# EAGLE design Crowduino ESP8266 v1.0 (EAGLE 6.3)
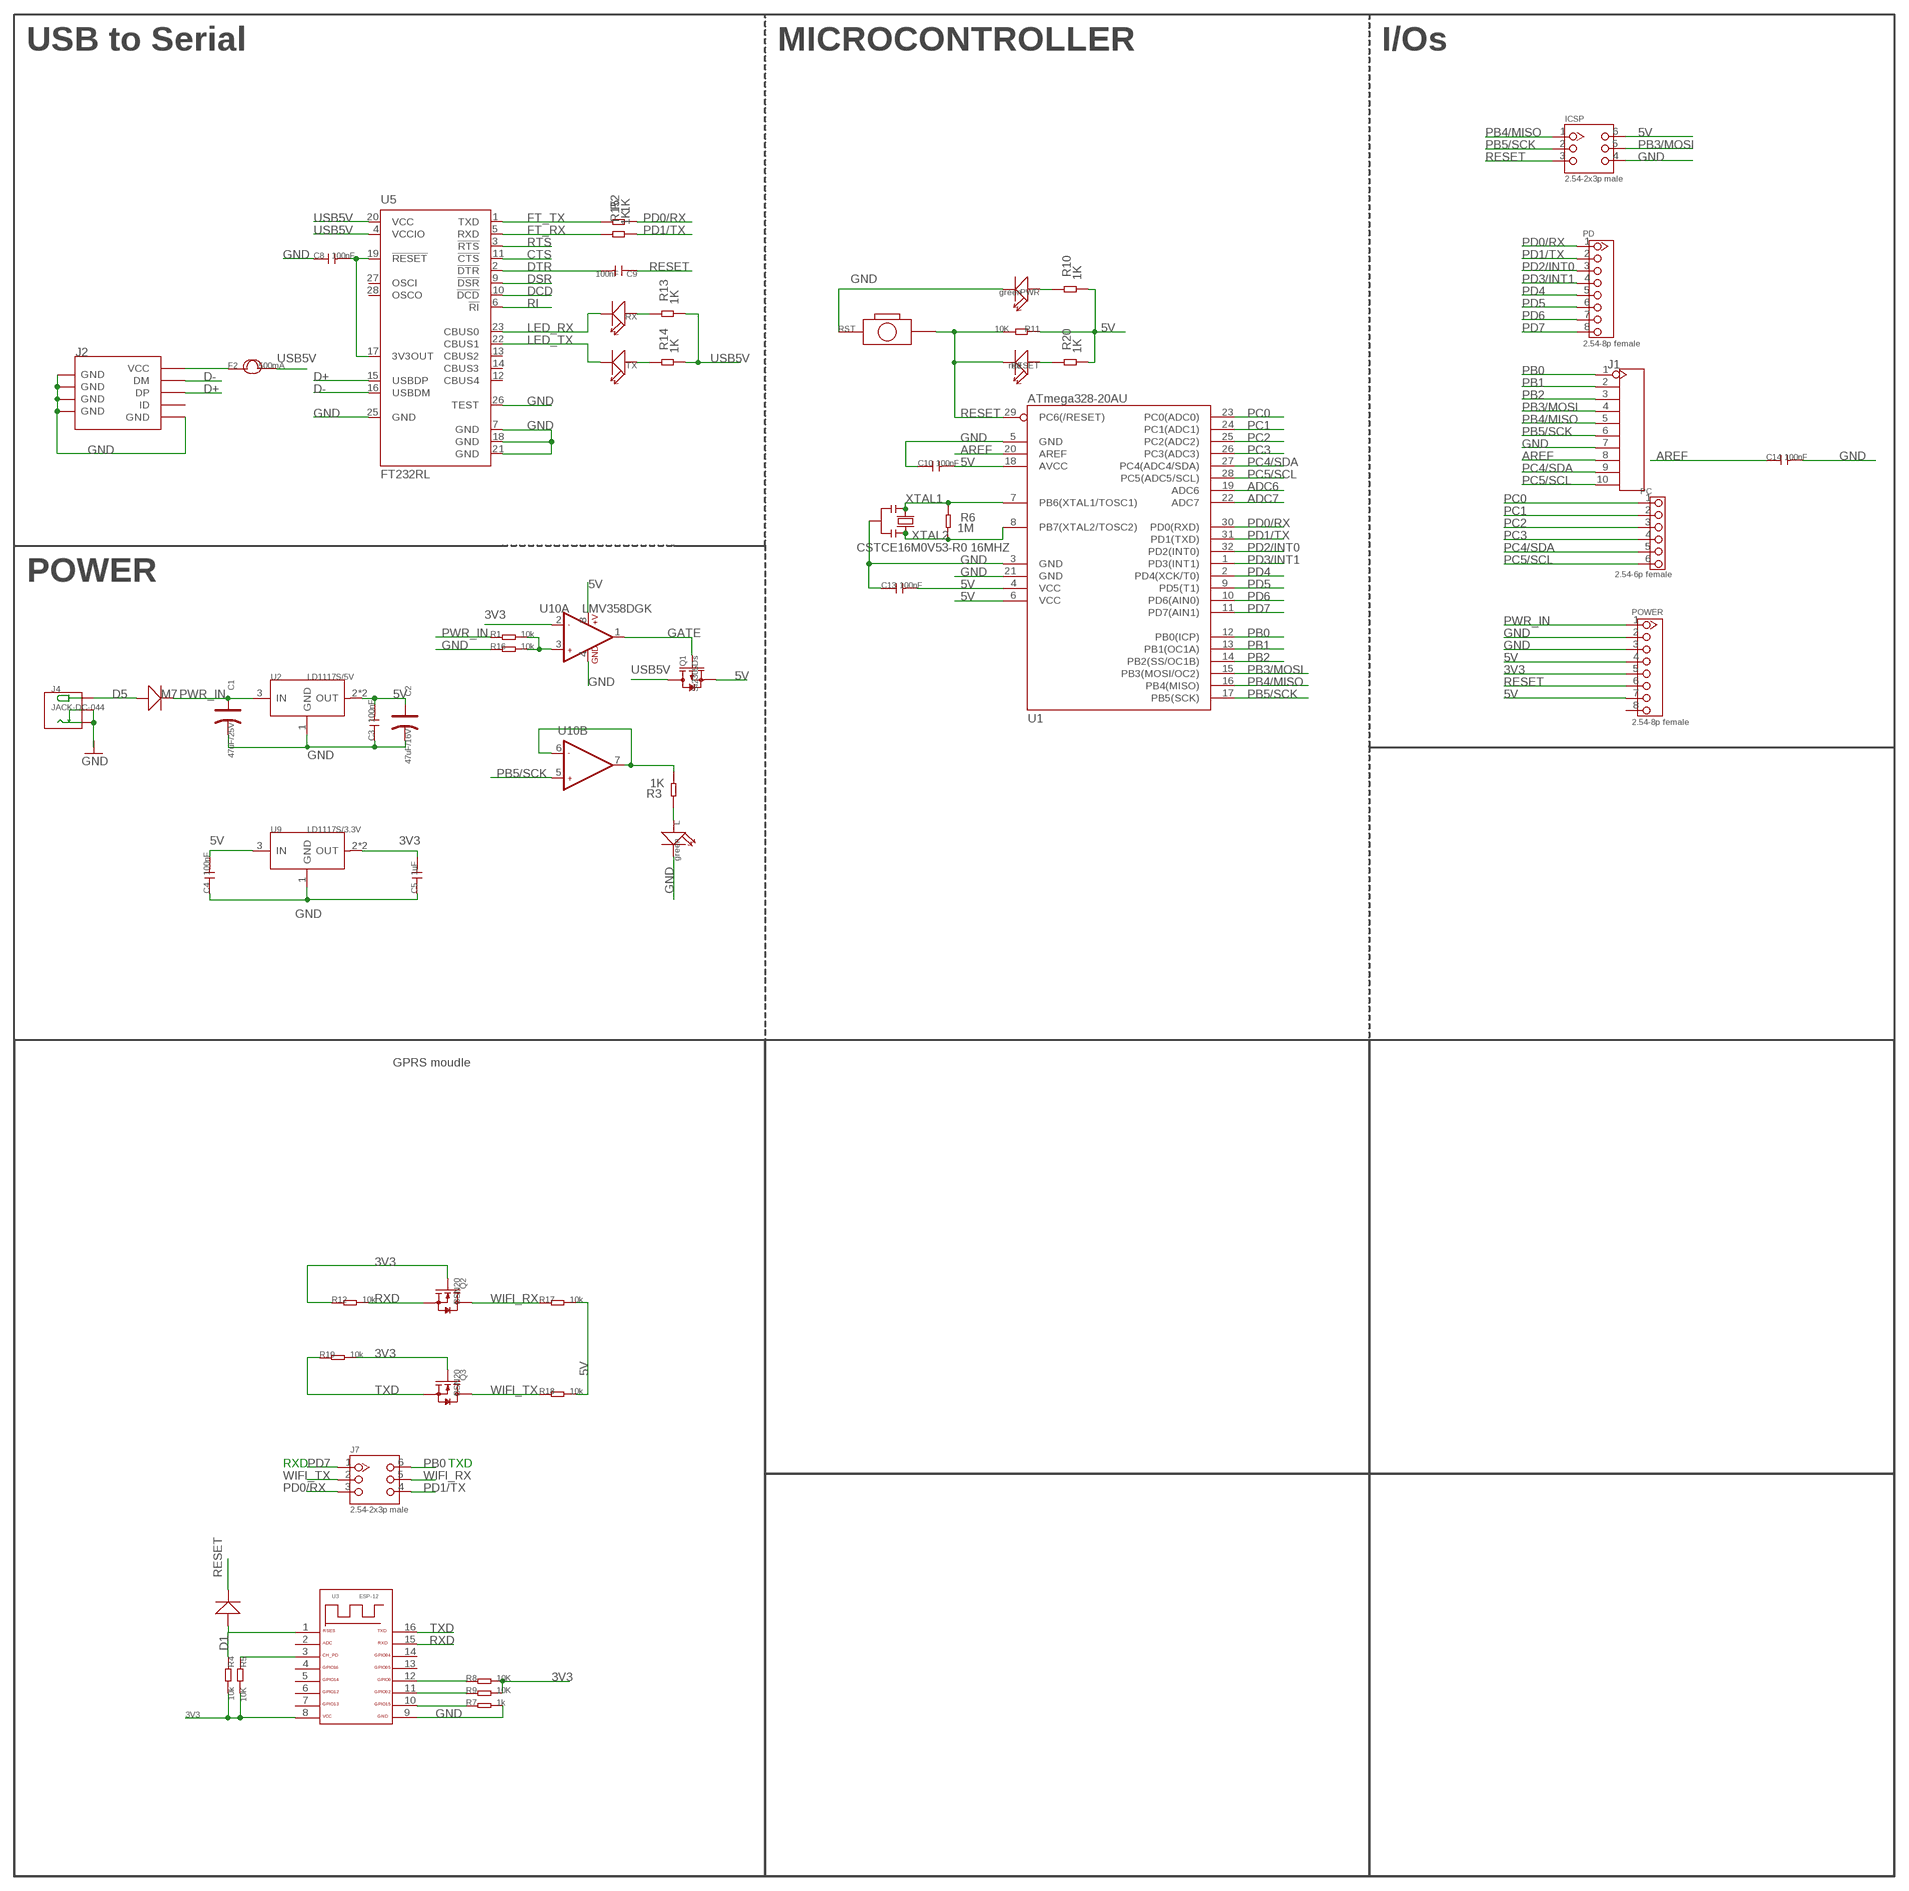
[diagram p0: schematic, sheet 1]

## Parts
C1  47uF/25V  CAP-AVX-C  [AVX-C]
C2  47uF/16V  CAP-AVX-A  [AVX-A]
C3  100nF  C-0603  [C0603]
C4  100nF  C-0603  [C0603]
C5  1uF  C-0603  [C0603]
C8  100nF  C-0603  [C0603]
C9  100nF  C-0603  [C0603]
C10  100nF  C-0603  [C0603]
C13  100nF  C-0603  [C0603]
C14  100nF  C-0603  [C0603]
D1  D'MBR0520LT1'  [SOD123-2.7X1.6]
D5  M7  D'SMA'  [D2010]
F2  500mA  FUSE1206  [R1206@1]
ICSP  2.54-2x3p male  HEADER-2X3P-2.54  [2X3P-2.54]
J1  HEADER-10P-2.54  [10P-2.54]
J2  USB-MINIUSB-5P-STRONG  [MINI-SMD-5P]
J4  JACK-DC-044  [DC-404]
J7  2.54-2x3p male  HEADER-2X3P-2.54  [2X3P-2.54]
L  green  LED'0603'  [LED-0603]
PC  2.54-6p female  HEADER-6P-65/35MIL  [6P-2.54-65/35MIL]
PD  2.54-8p female  HEADER-8P-2.54  [8P-2.54]
POWER  2.54-8p female  HEADER-8P-2.54  [8P-2.54]
PWR  green  LED'0603'  [LED-0603]
Q1  Si2305Ds  MOSFET-P'SI2323CDS/SI2305DS<BR>'  [SOT23@1]
Q2  BSN20  MOSFET-N'SOT23'  [SOT23]
Q3  BSN20  MOSFET-N'SOT23'  [SOT23]
R1  10k  R-0603  [R0603]
R2  1K  R-0603  [R0603]
R3  1K  R-0603  [R0603]
R4  10k  R-0603  [R0603]
R5  10K  R-0603  [R0603]
R6  1M  R-0603  [R0603]
R7  1k  R-0603  [R0603]
R8  10K  R-0603  [R0603]
R9  10K  R-0603  [R0603]
R10  1K  R-0603  [R0603]
R11  10K  R-0603  [R0603]
R12  10k  R-0603  [R0603]
R13  1K  R-0603  [R0603]
R14  1K  R-0603  [R0603]
R15  1K  R-0603  [R0603]
R16  10k  R-0603  [R0603]
R17  10k  R-0603  [R0603]
R18  10k  R-0603  [R0603]
R19  10k  R-0603  [R0603]
R20  1K  R-0603  [R0603]
RESET  red  LED'0603'  [LED-0603]
RST  BOTTON-2P-90D  [2P-7.62X3.56-90D]
RX  LED'0603'  [LED-0603]
TX  LED'0603'  [LED-0603]
U1  ATmega328-20AU  ATMEGA168  [TQFP32]
U2  LD1117S/5V  LD1117S  [SOT-223]
U3  ESP-12  [ESP-12]
U5  FT232RL  [SSOP28]
U9  LD1117S/3.3V  LD1117'SOT89'  [SOT89]
U10  LMV358DGK  [MSOP8]
Y2  CSTCE16M0V53-R0 16MHZ  RESONATORMU  [RESONATOR]

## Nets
3V3: C5.2 POWER.5 Q2.1(G) Q3.1(G) R4.2 R5.2 R8.2 R9.2 R12.1 R19.2 U3.8 U9.2(OUT) U9.4(OUT) U10.2(A:-IN1)
5V [usbvcc]: C2.+ C3.2 C4.2 C10.2 C13.2 ICSP.6 POWER.4 POWER.7 Q1.2(S) R10.1 R11.1 R17.2 R18.2 R20.1 U1.4(VCC) U1.6(VCC) U1.18(AVCC) U2.2(OUT) U2.TER(OUT) U9.3(IN) U10.8(A:+V)
ADC6: U1.19(ADC6)
ADC7: U1.22(ADC7)
AREF: C14.1 J1.8 U1.20(AREF)
CTS: U5.11(!CTS)
D+: J2.3(DP) U5.15(USBDP)
D-: J2.2(DM) U5.16(USBDM)
DCD: U5.10(!DCD)
DSR: U5.9(!DSR)
DTR: C9.2 U5.2(!DTR)
FT_RX: R15.2 U5.5(RXD)
FT_TX: R2.2 U5.1(TXD)
GATE: Q1.1(G) U10.1(A:OUT1)
GND: C1.- C2.- C3.1 C4.1 C5.1 C8.1 C10.1 C13.1 C14.2 ICSP.4 J1.7 J2.5(GND) J2.GND@1(GND) J2.GND@2(GND) J2.GND@3(GND) J2.GND@4(GND) J4.- J4.CDN L.- POWER.2 POWER.3 PWR.- R7.2 R16.1 RST.P$1 U1.3(GND) U1.5(GND) U1.21(GND) U2.1(GND) U3.9 U5.7(GND) U5.18(GND) U5.21(GND) U5.25(GND) U5.26(TEST) U9.1(GND) U10.4(A:GND) Y2.2
LED_RX: RX.- U5.23(CBUS0)
LED_TX: TX.- U5.22(CBUS1)
N$1: D5.+ J4.+
N$2: R13.2 RX.+
N$3: L.+ R3.2
N$4: R7.1 U3.10
N$5: R3.1 U10.6(B:-IN2) U10.7(B:OUT2)
N$6: C8.2 U5.17(3V3OUT) U5.19(!RESET)
N$7: PWR.+ R10.2
N$8: R14.2 TX.+
N$9: F2.1 J2.1(VCC)
N$10: R5.1 U3.3
N$11: D1.1(+) R4.1 U3.1
N$12: R8.1 U3.12
N$13: R9.1 U3.11
N$14: R1.2 R16.2 U10.3(A:+IN1)
N$15: R20.2 RESET.+
PB0: J1.1 J7.6 U1.12(PB0(ICP))
PB1: J1.2 U1.13(PB1(OC1A))
PB2: J1.3 U1.14(PB2(SS/OC1B))
PB3/MOSI: ICSP.5 J1.4 U1.15(PB3(MOSI/OC2))
PB4/MISO: ICSP.1 J1.5 U1.16(PB4(MISO))
PB5/SCK: ICSP.2 J1.6 U1.17(PB5(SCK)) U10.5(B:+IN2)
PC0: PC.1 U1.23(PC0(ADC0))
PC1: PC.2 U1.24(PC1(ADC1))
PC2: PC.3 U1.25(PC2(ADC2))
PC3: PC.4 U1.26(PC3(ADC3))
PC4/SDA: J1.9 PC.5 U1.27(PC4(ADC4/SDA))
PC5/SCL: J1.10 PC.6 U1.28(PC5(ADC5/SCL))
PD0/RX: J7.3 PD.1 R2.1 U1.30(PD0(RXD))
PD1/TX: J7.4 PD.2 R15.1 U1.31(PD1(TXD))
PD2/INT0: PD.3 U1.32(PD2(INT0))
PD3/INT1: PD.4 U1.1(PD3(INT1))
PD4: PD.5 U1.2(PD4(XCK/T0))
PD5: PD.6 U1.9(PD5(T1))
PD6: PD.7 U1.10(PD6(AIN0))
PD7: J7.1 PD.8 U1.11(PD7(AIN1))
PWR_IN: C1.+ D5.- POWER.1 R1.1 U2.3(IN)
RESET: C9.1 D1.2(-) ICSP.3 POWER.6 R11.2 RESET.- RST.P$2 U1.29(PC6(/RESET))
RI: U5.6(!RI)
RTS: U5.3(!RTS)
RXD: Q2.2(S) R12.2 U3.15
TXD: Q3.2(S) R19.1 U3.16
USB5V: F2.2 Q1.3(D) R13.1 R14.1 U5.4(VCCIO) U5.20(VCC)
WIFI_RX: J7.5 Q2.3(D) R17.1
WIFI_TX: J7.2 Q3.3(D) R18.1
XTAL1: R6.2 U1.7(PB6(XTAL1/TOSC1)) Y2.1
XTAL2: R6.1 U1.8(PB7(XTAL2/TOSC2)) Y2.3
Unconnected: J2.4(ID) POWER.8 U3.2 U3.4 U3.5 U3.6 U3.7 U3.13 U3.14 U5.12(CBUS4) U5.13(CBUS2) U5.14(CBUS3) U5.27(OSCI) U5.28(OSCO)

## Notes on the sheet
- USB to Serial | MICROCONTROLLER | I/Os
- POWER
- GPRS moudle
- RXD | TXD

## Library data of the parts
C1 C2 = Discrete:CAP*: Electrolytic Capacitors,Tantalum Capacitors and Super Capacitors
C3-C5 C8-C10 C13 C14 = Discrete:C*: Ceramic Capacitors
D1 D5 = Discrete:D*
F2 = Discrete:FUSE
ICSP J7 = Connector:HEADER-2X3P
J1 = Connector:HEADER-10P
J2 = Connector:USB-MINIUSB-5P
J4 = Connector:JACK-DC-044
L PWR RESET RX TX = Discrete:LED*
PC = Connector:HEADER-6P
PD POWER = Connector:HEADER-8P
Q1 = Discrete:MOSFET-P
Q2 Q3 = Discrete:MOSFET-N: IRLL014: http://www.vishay.com/docs/91319/sihll014.pdf
R1-R20 = Discrete:R*
RST = Discrete:BOTTON-2P
U1 = IC:ATMEGA168
U2 U9 = IC:LD1117: Low Drop Fixed And Adjustable Positive Voltage Regulators http://www.datasheetcatalog.org/datasheet/SGSThomsonMicroelectronics/mXuqtqv.pdf
U3 = Discrete:ESP-12
U5 = IC_SMD:FT232R: Source: http://www.ftdichip.com/Documents/DataSheets/DS_FT232R_v104.pdf
U10 = IC:LMV358: General purpose LOW Voltage, Rail-to-Rail Output Amplifiers http://www.fairchildsemi.com/ds/LM/LMV358.pdf
Y2 = SmartPrj:RESONATOR

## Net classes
0 default: clearance 0.152 mm
1 power: width 0.61 mm, drill 0.61 mm, clearance 0.254 mm
2 gnd: width 0.305 mm, drill 0.559 mm, clearance 0.254 mm
3 usbvcc: width 0.508 mm, drill 0.61 mm, clearance 0.254 mm

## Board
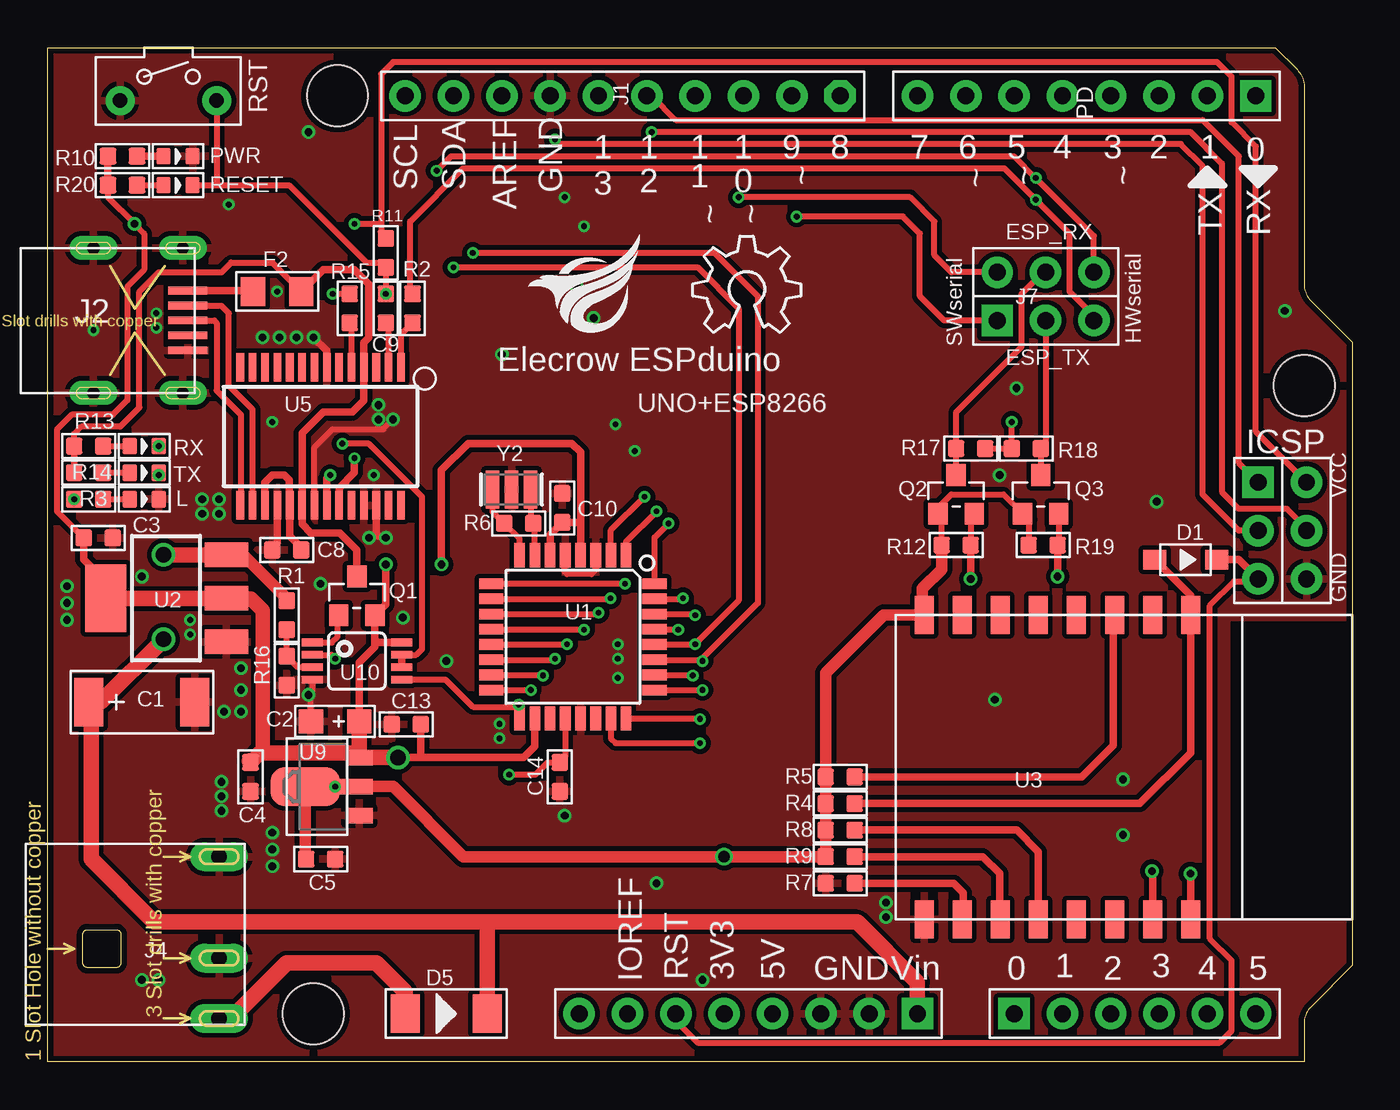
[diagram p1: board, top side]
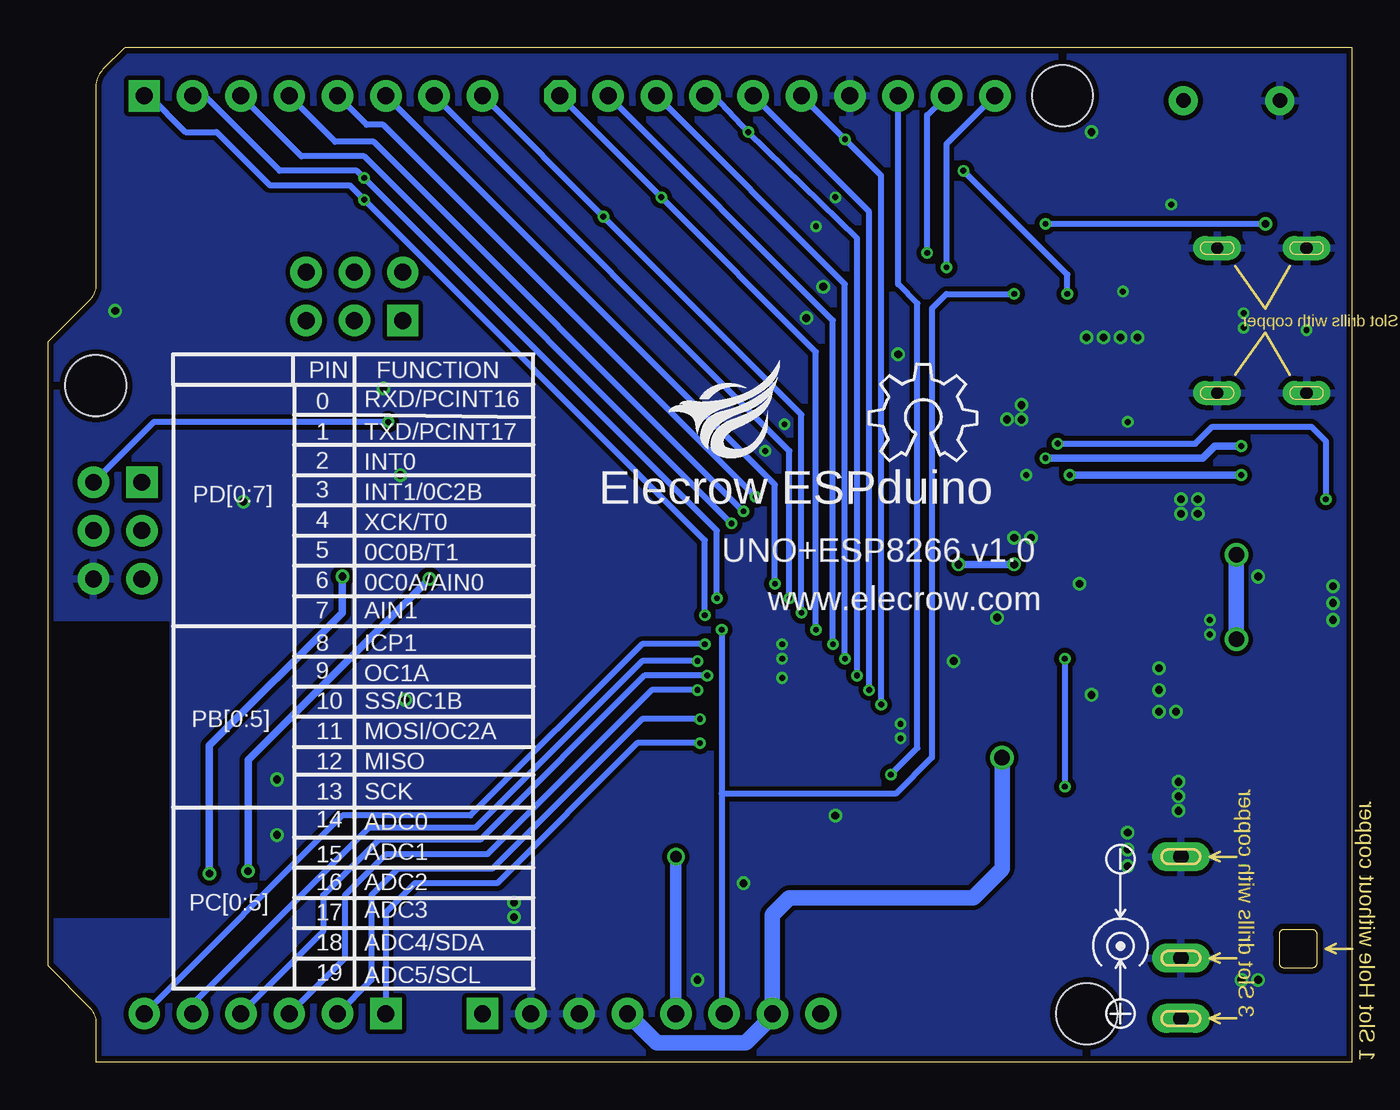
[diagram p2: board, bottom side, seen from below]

Size 68.58 x 53.34 mm. Coordinates in mm from the lower left corner, seen from the top.
Outline: 0,0 0,53.34 64.52,53.34 65.67,52.19 arc-45 66.04,51.29 66.04,40.91 arc45 66.41,40.01 68.58,37.85 68.58,5.08 66.41,2.91 arc45 66.04,2.01 66.04,0 0,0
Copper layers (1*16): Top 0.035mm / dielectric 1.5mm / Bottom 0.035mm
Design rules "MakerStudio *": minimum track width 6mil, minimum drill 10mil, track to track 6mil, track to pad 6mil, pad to pad 6mil, via to via 6mil, smd to smd 0mil, copper to edge 12mil, drill to drill 12mil, minimum pad ring 10mil, minimum via ring 6mil, stop-mask expansion 2mil, vias tented up to drill 100mil, thermal gap 10mil
Holes 3.2 mm at 15.24,50.8 66.04,35.56 13.97,2.54

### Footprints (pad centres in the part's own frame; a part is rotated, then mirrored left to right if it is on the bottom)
AVX-C = smd 1.524 x 2.54: + -2.794,0; - 2.794,0
AVX-A = smd 1.27 x 1.27: + -1.27,0; - 1.27,0
C0603 = smd 0.889 x 0.889: 1 -0.762,0; 2 0.762,0
SOD123-2.7X1.6 = smd 1.2 x 1.02: 1 -1.635,0; 2 1.635,0
D2010 = smd 1.524 x 2.032: + -2.159,0; - 2.159,0
R1206@1 = smd 1.27 x 1.524: 1 -1.27,0; 2 1.27,0
2X3P-2.54 = drill 0.889 pad 1.651 square: 1 -1.27,2.54 | drill 0.889 pad 1.651: 2 -1.27,0; 3 -1.27,-2.54; 4 1.27,-2.54; 5 1.27,0; 6 1.27,2.54
10P-2.54 = drill 0.889 pad 1.651 octagon: 1 0,11.43 | drill 0.889 pad 1.651: 2 0,8.89; 3 0,6.35; 4 0,3.81; 5 0,1.27; 6 0,-1.27; 7 0,-3.81; 8 0,-6.35; 9 0,-8.89; 10 0,-11.43
MINI-SMD-5P = smd 2.032 x 0.406: 1 0.381,-1.575; 2 0.381,-0.787; 3 0.381,0; 4 0.381,0.787; 5 0.381,1.575 | drill 0.635 pad 1.27 long: GND@1 0.635,3.81; GND@2 5.334,3.81; GND@3 5.334,-3.81; GND@4 0.635,-3.81
DC-404 = drill 0.813 pad 1.524 long: + 3.175,10.16; - -5.334,10.16; CDN 0,10.16
LED-0603 = smd 0.762 x 0.889: + -0.762,0; - 0.762,0
6P-2.54-65/35MIL = drill 0.889 pad 1.651 square: 1 0,6.35 | drill 0.889 pad 1.651: 2 0,3.81; 3 0,1.27; 4 0,-1.27; 5 0,-3.81; 6 0,-6.35
8P-2.54 = drill 0.889 pad 1.651 square: 1 0,8.89 | drill 0.889 pad 1.651: 2 0,6.35; 3 0,3.81; 4 0,1.27; 5 0,-1.27; 6 0,-3.81; 7 0,-6.35; 8 0,-8.89
SOT23@1 = smd 1.016 x 1.143: 1 -0.95,-1.016; 2 0.95,-1.016; 3 0,1.016
SOT23 = smd 1.016 x 1.143: 1 -0.95,-1.016; 2 0.95,-1.016; 3 0,1.016
R0603 = smd 0.889 x 0.889: 1 -0.762,0; 2 0.762,0
2P-7.62X3.56-90D = drill 0.762 pad 1.524: P$1 0,2.54; P$2 0,-2.54
TQFP32 = smd 1.27 x 0.559: 1 -4.293,2.8; 2 -4.293,2; 3 -4.293,1.2; 4 -4.293,0.4; 5 -4.293,-0.4; 6 -4.293,-1.2; 7 -4.293,-2; 8 -4.293,-2.8; 17 4.293,-2.8; 18 4.293,-2; 19 4.293,-1.2; 20 4.293,-0.4; 21 4.293,0.4; 22 4.293,1.2; 23 4.293,2; 24 4.293,2.8 | smd 0.559 x 1.27: 9 -2.8,-4.293; 10 -2,-4.293; 11 -1.2,-4.293; 12 -0.4,-4.293; 13 0.4,-4.293; 14 1.2,-4.293; 15 2,-4.293; 16 2.8,-4.293; 25 2.8,4.293; 26 2,4.293; 27 1.2,4.293; 28 0.4,4.293; 29 -0.4,4.293; 30 -1.2,4.293; 31 -2,4.293; 32 -2.8,4.293
SOT-223 = smd 1.27 x 2.286: 1 -2.286,-3.175; 2 0,-3.175; 3 2.286,-3.175 | smd 3.556 x 2.159: TER 0,3.175
ESP-12 = smd 2 x 1: 1 0,15.5; 2 0,13.5; 3 0,11.5; 4 0,9.5; 5 0,7.5; 6 0,5.5; 7 0,3.5; 8 0,1.5; 9 16,1.5; 10 16,3.5; 11 16,5.5; 12 16,7.5; 13 16,9.5; 14 16,11.5; 15 16,13.5; 16 16,15.5
SSOP28 = smd 0.4 x 1.5: 1 -4.225,-3.625; 2 -3.575,-3.625; 3 -2.925,-3.625; 4 -2.275,-3.625; 5 -1.625,-3.625; 6 -0.975,-3.625; 7 -0.325,-3.625; 8 0.325,-3.625; 9 0.975,-3.625; 10 1.625,-3.625; 11 2.275,-3.625; 12 2.925,-3.625; 13 3.575,-3.625; 14 4.225,-3.625; 15 4.225,3.625; 16 3.575,3.625; 17 2.925,3.625; 18 2.275,3.625; 19 1.625,3.625; 20 0.975,3.625; 21 0.325,3.625; 22 -0.325,3.625; 23 -0.975,3.625; 24 -1.625,3.625; 25 -2.275,3.625; 26 -2.925,3.625; 27 -3.575,3.625; 28 -4.225,3.625
SOT89 = smd 0.8 x 1.4: 1 -1.524,-1.905; 3 1.524,-1.905 | smd 0.8 x 1.9: 2 0,-1.651 | smd 2.032 x 3.65: 4 0,0.94
MSOP8 = smd 0.4 x 1.1: 1 -0.975,-2.35; 2 -0.325,-2.35; 3 0.325,-2.35; 4 0.975,-2.35; 5 0.975,2.35; 6 0.325,2.35; 7 -0.325,2.35; 8 -0.975,2.35
RESONATOR = smd 0.7 x 2: 1 -1,0; 2 0,0; 3 1,0

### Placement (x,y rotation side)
C1  4.95,18.92 0 top
C2  15.11,17.91 180 top
C3  2.67,27.56 180 top
C4  10.67,14.99 90 top
C5  14.35,10.67 180 top
C8  12.57,26.92 0 top
C9  17.78,39.62 270 top
C10  27.05,29.13 270 top
C13  18.85,17.75 0 top
C14  26.92,14.99 270 top
D1  59.82,26.42 0 top
D5  20.95,2.54 0 top
F2  12.06,40.51 0 top
ICSP  64.9,27.94 0 top
J1  30.23,50.8 270 top
J2  7.75,38.99 180 top
J4  -1.14,5.46 270 top
J7  52.45,40.26 90 top
L  5.08,29.59 0 top
PC  57.15,2.54 90 top
PD  54.61,50.8 270 top
POWER  36.83,2.54 270 top
PWR  6.86,47.62 0 top
Q1  16.26,24.51 0 top
Q2  47.75,29.84 0 top
Q3  52.2,29.84 0 top
R1  12.57,23.5 270 top
R2  19.18,39.62 270 top
R3  2.16,29.59 0 top
R4  41.66,13.59 180 top
R5  41.66,14.99 180 top
R6  24.77,28.32 0 top
R7  41.66,9.4 180 top
R8  41.66,12.19 180 top
R9  41.66,10.79 180 top
R10  3.94,47.62 0 top
R11  17.78,42.55 270 top
R12  47.75,27.18 0 top
R13  2.16,32.38 0 top
R14  2.16,30.99 0 top
R15  15.88,39.62 270 top
R16  12.57,20.57 90 top
R17  48.51,32.26 0 top
R18  51.44,32.26 180 top
R19  52.32,27.18 180 top
R20  3.94,46.1 0 top
RESET  6.86,46.1 0 top
RST  6.35,50.55 90 top
RX  5.08,32.38 0 top
TX  5.08,30.99 0 top
U1  27.61,22.35 270 top
U2  6.22,24.38 90 top
U3  44.58,23.5 270 top
U5  14.35,32.89 180 top
U9  14.48,14.48 90 top
U10  16.26,21.08 270 top
U$1  [ELECROW_NEW_4]  35.94,31.75 0 bottom
U$2  [ELECROW_NEW_4]  25.27,38.35 0 top
U$4  [OSHW_6X200_NOTEXT]  33.91,38.35 0 top
U$5  [OSHW_6X200_NOTEXT]  25.4,31.62 0 bottom
Y2  24.38,30.1 180 top

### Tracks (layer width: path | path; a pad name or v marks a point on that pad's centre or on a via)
3V3  (via drill 0.3, 0.61)
  Top 0.305: U10.2 14.91,21.41 v15.11,21.21 | R12.1 46.99,28.64 Q2.1 46.8,29.15 47.5,29.84 50.23,29.84 Q3.1 | 51.56,28.51 R19.2
  Top 0.406: 51.56,28.51 Q3.1
  Top 0.61: R12.1 46.99,25.91 45.97,24.89 45.97,23.6 U3.8 43.94,23.5 40.89,20.45 R5.2 R4.2 R8.2 R9.2 v35.56,10.79 21.84,10.79 18.16,14.48 U9.2 v15.11,14.48 U9.4 13.54,10.72 C5.2
  Bottom 0.305: v15.11,21.21 v15.11,14.48
  Bottom 0.61: v35.56,10.79 POWER.5
5V  (via drill 0.3, 0.41, 0.81)
  Top 0.305: C3.2 0.51,28.96 0.51,33.27 1.27,34.04 3.43,34.04 4.19,34.8 4.19,40.77 5.08,41.66 5.08,43.56 v4.57,44.07 3.17,45.47 R20.1 | R17.2 R18.2 v50.67,33.66 | ICSP.6 63.5,33.15 63.5,48.13 62.23,49.4 62.23,51.82 61.47,52.58 18.16,52.58 17.53,51.94 17.53,44.07 | 17.53,44.07 17.53,43.56 R11.1 | v16.13,44.07 17.53,44.07
  Top 0.406: C2.+ 16.38,21 17.21,21.82 17.21,22.23 | U2.TER 3.05,25.27 1.91,26.42 C3.2 | 19.56,16 25.02,16 25.61,16.59 U1.18 | 19.56,16 v18.41,16 | C13.2 19.61,16.05 19.56,16 | v17.78,26.16 17.78,24.07 Q1.2 17.21,22.23 | U10.8 17.37,22.06 17.21,22.23 | U1.4 28.01,28.32 | 28.01,28.32 28.01,32.06 27.56,32.51 22.1,32.51 20.7,31.11 v20.7,26.16 | U1.6 26.41,27.73 C10.2 27.96,28.37 28.01,28.32 | R10.1 R20.1
  Top 0.762: U2.2 10.67,24.38 11.3,23.75 11.3,16.38 11.05,16.13 C4.2
  Top 0.813: 10.59,15.82 C4.2 | U9.3 C2.+ | U2.TER U2.2 | 11.05,16.13 11.18,16.26 16.13,16.26 U9.3 | U9.3 v18.41,16
  Bottom 0.305: v50.67,33.66 62.99,33.66 ICSP.6 | v16.13,44.07 v4.57,44.07
  Bottom 0.406: v20.7,26.16 v17.78,26.16
  Bottom 0.61: POWER.7 30.48,2.41
  Bottom 0.813: v18.41,16 18.41,10.16 19.94,8.64 29.59,8.64 30.48,7.75 POWER.7 | 30.48,2.41 31.88,1.02 36.58,1.02 POWER.4
AREF  (via drill 0.3)
  Top 0.305: U1.20 27.21,16.09 C14.1 26.29,15.75 25.65,15.11 v24.26,15.11
  Bottom 0.305: v24.26,15.11 22.86,16.51 22.86,39.88 23.88,40.89 J1.8
D+
  Top 0.305: J2.3 8.76,38.99 8.89,38.86 8.89,35.31 10.16,34.04 10.16,29.3 U5.15
D-
  Top 0.305: U5.16 10.78,34.31 9.53,35.56 9.53,39.37 9.14,39.75 7.39,39.75 J2.2
DTR
  Top 0.305: U5.2 17.93,38.72 C9.2
FT_RX
  Top 0.305: U5.5 15.98,38.76 R15.2
FT_TX
  Top 0.305: U5.1 18.58,38.26 R2.2
GATE
  Top 0.305: U10.1 14.95,22.06 15.24,22.35 15.24,23.43 Q1.1
GND  (via drill 0.3, 0.41)
  Top 0.305: U1.3 28.81,25.89 28.57,25.65 27.3,25.65 27.18,25.78 27.18,26.61 U1.5 | U5.21 14.03,32.31 14.99,33.27 17.65,33.27 v18.16,33.78 | C2.- 13.84,19.18 v13.72,19.3 13.91,19.49 U10.4
  Top 0.406: U5.18 12.08,27.32 C8.1 | U5.26 17.28,27.68 v17.78,27.56 | U5.7 14.68,37.39 v13.97,38.1
  other vias: 11.81,33.66 9.02,29.59 5.71,39.37 5.71,38.61 12.06,40.51 9.53,45.09 4.95,25.53 2.41,38.48 18.67,23.37 29.97,21.21 29.97,20.19 23.75,17.02 23.75,17.78 1.02,25.02 1.02,24.13 7.49,23.24 7.49,22.48 10.16,19.56 10.16,18.41 16.89,27.56 13.08,38.1 12.19,38.1 11.3,38.1 17.4,33.78 17.4,34.54 20.95,21.08 14.35,25.15 10.16,20.7 9.27,18.41 9.14,14.73 9.14,13.97 9.14,13.21 11.81,12.06 11.81,11.18 11.81,10.29 1.02,23.24 9.02,28.83 8.13,29.59 8.13,28.83 29.97,21.97 5.84,4.32 32,9.4 27.18,12.95 4.95,4.32 34.42,4.32 13.72,48.9 50.93,35.43 50.04,30.86 23.88,37.21 28.7,39.12 27.81,40.77 28.19,43.94 27.18,45.47 29.84,33.53 30.86,32.13 17.14,30.86 49.78,19.05 58.29,29.46 56.52,11.94 56.52,14.86 65.02,39.5 44.07,8.38 44.07,7.62
  pour Top (isolate 0.254): 0,0 68.71,0 68.71,7.37 61.98,7.37 61.98,23.37 69.85,23.37 69.85,53.34 0,53.34
  pour Bottom (isolate 0.254): 0,0 68.71,0 68.71,7.37 61.98,7.37 61.98,23.37 69.85,23.37 69.85,53.34 0,53.34
LED_RX  (via drill 0.3)
  Top 0.406: U5.23 15.33,30.18 16.13,30.99 v16.13,31.75
  Bottom 0.406: v16.13,31.75 7.87,31.75 7.24,32.38 RX.-
  other vias: 5.84,32.38
LED_TX  (via drill 0.3)
  Top 0.406: v5.84,30.86 5.97,30.86 TX.- | U5.22 14.68,30.68 v14.86,30.86
  Bottom 0.406: v14.86,30.86 v5.84,30.86
N$1
  Top 0.813: J4.+ 9.65,2.29 12.57,5.21 17.27,5.21 18.8,3.68 D5.+
N$2
  Top 0.305: R13.2 RX.+
N$3
  Top 0.305: R3.2 L.+
N$4
  Top 0.406: R7.1 47.62,9.4 48.13,8.89 48.13,7.55 U3.10
N$5  (via drill 0.3)
  Top 0.305: U10.7 19.38,21.41 19.68,21.72 19.68,29.72 16.89,32.51 v15.49,32.51
  Top 0.406: U10.7 U10.6
  Bottom 0.305: v15.49,32.51 8.26,32.51 7.37,33.4 2.16,33.4 1.4,32.64 R3.1
  other vias: 1.4,29.59
N$6
  Top 0.406: U5.17 11.43,30.48 11.81,30.86 12.45,30.86 12.7,30.61 12.7,29.29 U5.19 12.73,27.66 13.34,27.05 C8.2
N$7
  Top 0.406: R10.2 PWR.+
N$8
  Top 0.305: R14.2 TX.+
N$9
  Top 0.406: J2.1 10.74,40.56 F2.1
N$10
  Top 0.406: R5.1 54.36,14.99 56.01,16.64 56.01,23.43 U3.3
N$11
  Top 0.406: R4.1 57.4,13.59 60.07,16.26 U3.1 60.08,24.52 D1.1
N$12
  Top 0.406: R8.1 50.93,12.19 52.07,11.05 U3.12
N$13
  Top 0.406: R9.1 49.15,10.79 50.04,9.91 50.04,7.53 U3.11
N$14
  Top 0.305: U10.3 13.15,20.76 R16.2 R1.2
N$15
  Top 0.305: R20.2 RESET.+
PB0  (via drill 0.3)
  Top 0.305: U1.12 28.18,22.75 v28.19,22.73 | J7.6 47.5,41.53 46.61,42.42 46.61,44.2 45.34,45.47 v36.32,45.47
  Bottom 0.305: 41.66,50.67 J1.1 36.39,45.53 | v28.19,22.73 28.19,37.34 36.39,45.53 | v36.32,45.47 36.45,45.47 36.39,45.53
PB1  (via drill 0.3)
  Top 0.305: U1.13 27.29,21.95 v27.3,21.97
  Bottom 0.305: v27.3,21.97 27.3,38.99 J1.2
PB2  (via drill 0.3)
  Top 0.305: U1.14 26.61,21.15 v26.67,21.21
  Bottom 0.305: v26.67,21.21 26.67,40.89 J1.3
PB3/MOSI  (via drill 0.3)
  Top 0.305: U1.15 26,20.35 v26.04,20.32 | v31.75,48.9 60.07,48.9 61.72,47.24 61.72,29.97 62.61,29.08 65.15,29.08 66.17,28.07 ICSP.5
  Bottom 0.305: v26.04,20.32 26.04,43.31 v31.75,48.9 33.53,50.8 J1.4
PB4/MISO  (via drill 0.3)
  Top 0.305: U1.16 v25.39,19.55 v25.4,19.56 | J1.5 31.75,50.8 33.02,49.53 60.71,49.53 62.61,47.62 62.61,31.5 ICSP.1
  Bottom 0.305: v25.4,19.56 25.4,44.7 J1.5
PB5/SCK  (via drill 0.3)
  Top 0.305: U1.17 24.77,18.1 v24.77,18.8 24.64,18.67 22.35,18.67 20.91,20.11 U10.5 | v26.67,48.51 26.92,48.26 59.56,48.26 60.71,47.12 60.71,29.84 62.61,27.94 ICSP.2
  Bottom 0.305: v24.77,18.8 24.77,46.61 v26.67,48.51 J1.6
PC0  (via drill 0.3)
  Top 0.305: U1.23 29.61,17 29.84,16.76 v34.29,16.76
  Bottom 0.305: v34.29,16.76 37.59,16.76 44.96,9.4 49.28,9.4 50.8,7.87 PC.1
PC1  (via drill 0.3)
  Top 0.305: U1.24 34.27,18.06 v34.29,18.03
  Bottom 0.305: v34.29,18.03 37.34,18.03 45.21,10.16 50.16,10.16 51.56,8.76 51.56,4.32 PC.2
PC2  (via drill 0.3)
  Top 0.305: U1.25 v34.41,19.55 v34.42,19.56
  Bottom 0.305: v34.42,19.56 36.83,19.56 45.47,10.92 50.8,10.92 52.96,8.76 52.96,5.46 PC.3
PC3  (via drill 0.3)
  Top 0.305: U1.26 33.88,20.35 v33.91,20.32
  Bottom 0.305: v33.91,20.32 37.21,20.32 45.85,11.68 51.18,11.68 54.1,8.76 54.1,6.86 PC.4
PC4/SDA  (via drill 0.3)
  Top 0.305: U1.27 34.35,21.15 v34.42,21.08 34.42,21.21 37.34,24.13 37.34,40.26 35.05,42.55 v22.35,42.55
  Bottom 0.305: v34.42,21.08 37.34,21.08 46.1,12.32 51.69,12.32 60.71,3.3 60.71,2.79 PC.5 | v22.35,42.55 22.35,49.78 J1.9
PC5/SCL  (via drill 0.3)
  Top 0.305: U1.28 34.02,21.95 v34.04,21.97 36.32,24.26 36.32,39.62 34.16,41.78 v21.34,41.78
  Bottom 0.305: v34.04,21.97 37.34,21.97 46.35,12.95 53.09,12.95 PC.6 | J1.10 21.34,48.26 v21.34,41.78
PD0/RX  (via drill 0.3)
  Top 0.305: U1.30 33.85,23.55 v34.04,23.5 | R2.1 19.05,40.51 19.05,44.2 21.84,46.99 50.29,46.99 v51.94,45.34 53.72,43.56 53.72,40.51 54.99,39.24 J7.3
  Bottom 0.305: PD.1 63.25,50.8 61.34,48.9 59.69,48.9 56.9,46.1 52.7,46.1 v51.94,45.34 34.04,27.43 v34.04,23.5
PD1/TX  (via drill 0.3)
  Top 0.305: R15.1 v14.99,40.39 | v20.45,46.86 21.21,47.62 50.8,47.62 v51.94,46.48 54.99,43.43 J7.4 | U1.31 33.37,24.35 v33.4,24.38
  Bottom 0.305: PD.2 60.33,50.8 56.39,46.86 52.32,46.86 v51.94,46.48 33.4,27.94 v33.4,24.38 | v14.99,40.39 14.99,41.4 v20.45,46.86
PD2/INT0  (via drill 0.3)
  Top 0.305: U1.32 31.9,27.58 v32.64,28.32
  Bottom 0.305: PD.3 55.24,47.62 51.94,47.62 v32.64,28.32
PD3/INT1  (via drill 0.3)
  Top 0.305: U1.1 30.41,27.36 v32,28.96
  Bottom 0.305: PD.4 53.47,48.39 51.44,48.39 v32,28.96
PD4  (via drill 0.3)
  Top 0.305: U1.2 29.61,27.96 v31.37,29.72
  Bottom 0.305: v31.37,29.72 50.93,49.28 51.82,49.28 PD.5
PD5  (via drill 0.3)
  Top 0.305: U1.9 v30.35,25.15
  Bottom 0.305: v30.35,25.15 30.35,30.35 PD.6
PD6  (via drill 0.3)
  Top 0.305: U1.10 29.56,24.35 v29.59,24.38
  Bottom 0.305: v29.59,24.38 29.59,32.13 PD.7
PD7  (via drill 0.3)
  Top 0.305: U1.11 28.89,23.55 v28.96,23.62 | J7.1 47.12,38.99 45.85,40.26 45.85,43.56 44.96,44.45 v39.37,44.45
  Bottom 0.305: v28.96,23.62 28.96,34.04 v39.37,44.45 PD.8
PWR_IN  (via drill 0.81)
  Top 0.61: R1.1 12.57,24.38 10.29,26.67 U2.3
  Top 0.813: v6.1,22.23 2.79,18.92 C1.+ 2.29,18.8 2.29,10.67 5.59,7.37 23.37,7.37 | v6.1,26.67 U2.3 | POWER.1 45.72,4.19 42.55,7.37 23.37,7.37 | D5.- 23.11,7.11 23.37,7.37
  Bottom 0.813: v6.1,22.23 v6.1,26.67
RESET  (via drill 0.3)
  Top 0.305: POWER.6 33.02,2.16 34.16,1.02 61.59,1.02 62.23,1.65 62.23,5.33 61.09,6.48 61.09,24 62.36,25.27 63.5,25.27 ICSP.3 | U1.29 33.13,22.75 v33.15,22.73 | C9.1 R11.2 17.53,42.04 16.76,42.04 12.7,46.1 9.02,46.1 | RESET.- 9.02,46.1 | RST.P$2 8.89,46.23 9.02,46.1
  Top 0.406: D1.2 62.61,26.42 ICSP.3
  Bottom 0.305: v33.15,22.73 33.15,14.1 | 33.15,14.1 33.15,2.67 POWER.6 | 33.15,14.1 24,14.1 22.1,16 22.1,39.62 21.34,40.39 C9.1
  other vias: 17.78,40.39
RXD  (via drill 0.41)
  Top 0.305: 48.51,28.64 R12.2
  Top 0.406: 48.51,28.64 Q2.2 | U3.15 58.08,9.99 v58.04,10.03 | v48.51,25.4 R12.2
  Bottom 0.406: v58.04,10.03 58.04,15.88 v48.51,25.4
TXD  (via drill 0.41)
  Top 0.305: Q3.2 53.15,27.24 R19.1
  Top 0.406: U3.16 v60.08,9.9 v60.07,9.91 | v53.09,25.53 R19.1
  Bottom 0.406: v60.07,9.91 60.07,16.64 53.09,23.62 v53.09,25.53
USB5V
  Top 0.305: R13.1 R14.1 1.4,33.02 1.78,33.4 3.81,33.4 4.83,34.42 4.83,40.51 5.84,41.53 9.14,41.53 9.65,42.04 11.81,42.04 F2.2
  Top 0.406: F2.2 14.48,41.66 16.13,41.66 16.89,40.89 16.89,38.1 16.63,37.84 U5.4 16.63,34.79 16,34.16 14.48,34.16 13.38,33.06 U5.20 13.38,28.28 13.84,27.81 15.37,27.81 16.26,26.92 Q1.3
WIFI_RX
  Top 0.305: Q2.3 R17.1 47.75,34.16 51.18,37.59 51.18,40.39 52.32,41.53 J7.5
WIFI_TX
  Top 0.305: J7.2 52.45,32.51 R18.1 Q3.3
XTAL1
  Top 0.305: U1.7 25.61,28.24 R6.2 25.38,28.46 Y2.1
XTAL2
  Top 0.305: Y2.3 23.38,28.94 R6.1 24.81,27.51 U1.8

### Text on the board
tPlace: 1 | 1 | 1 | 1 | 9 | 8 | 7 | 6 | 5 | 4 | 3 | 2 | 1 | 0 | SCL | SDA | GND | 3 | 2 | 1 | 0 | ~ | ~ | ~ | ~ | AREF | ~ | ~ | ESP_RX | SWserial | HWserial | ESP_TX | Elecrow ESPduino | UNO+ESP8266 | VCC | GND | IOREF | RST | 3V3 | 5V | GND | Vin | 0 | 1 | 2 | 3 | 4 | 5
bPlace: PIN | FUNCTION | RXD/PCINT16 | 0 | 1 | INT0 | TXD/PCINT17 | 2 | INT1/0C2B | 3 | Elecrow ESPduino | PD[0:7] | XCK/T0 | 4 | UNO+ESP8266 v1.0 | 0C0B/T1 | 5 | 0C0A/AIN0 | 6 | www.elecrow.com | AIN1 | 7 | ICP1 | 8 | OC1A | 9 | SS/0C1B | 10 | PB[0:5] | MOSI/OC2A | 11 | MISO | 12 | SCK | 13 | ADC0 | 14 | ADC1 | 15 | ADC2 | 16 | ADC3 | PC[0:5] | 17 | ADC4/SDA | 18 | ADC5/SCL | 19
tNames: TX | RX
